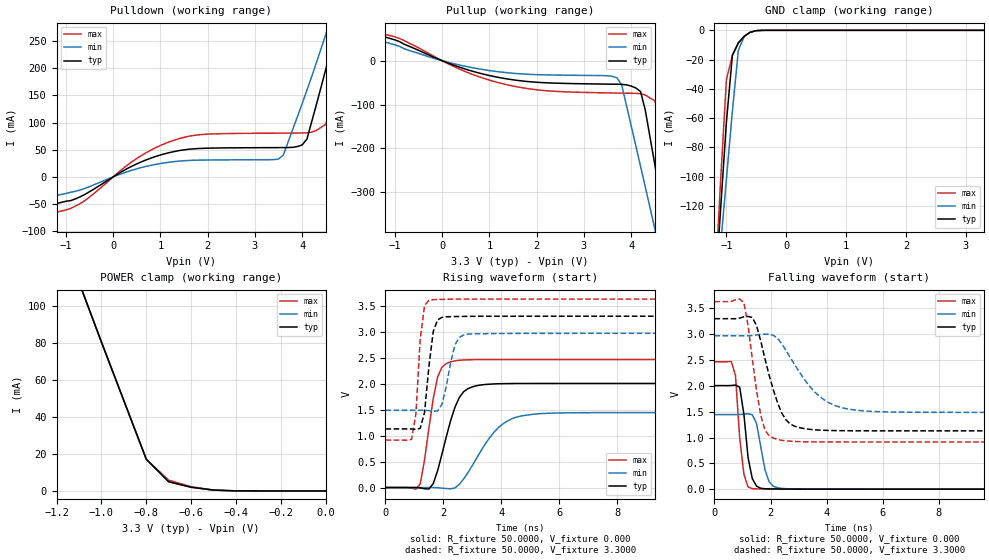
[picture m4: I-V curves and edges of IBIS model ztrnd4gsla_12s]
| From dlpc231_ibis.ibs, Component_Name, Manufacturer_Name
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| Model ztrnd4gsla_12s
[Model]   ztrnd4gsla_12s
Model_type   I/O
Polarity   Non-Inverting
Enable   Active-High
Vinl = 0.8000V
Vinh = 2.0000V
Vmeas = 1.5000V
Cref =50.0000pF
Rref = 0.5000k
Vref =  0.000V
C_comp   0.7000pF   0.7000pF   0.7000pF
[Temperature Range]   25.0000   0.1240k   -40.0000
[Voltage Range]   3.3000V   2.9700V   3.6300V
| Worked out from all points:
|   slope of the pulldown table from 0 to 0.495 V, typ, clamps not added: 20.8 ohm
|   slope of the pullup table from 0 to 0.495 V, typ, clamps not added: 25.7 ohm
|   GND clamp passes 1 mA (typ) near -0.57 V on its own axis
|   POWER clamp passes 1 mA (typ) near -0.54 V on its own axis
|   rising waveform, R_fixture 50.0000, V_fixture 0.000: 20-80 % time 609ps typ, 1.05ns min, 408ps max; typ from 0 V to 2 V
|   rising waveform, R_fixture 50.0000, V_fixture 3.3000: 20-80 % time 249ps typ, 339ps min, 199ps max; typ from 1.13 V to 3.3 V
|   falling waveform, R_fixture 50.0000, V_fixture 0.000: 20-80 % time 270ps typ, 317ps min, 228ps max; typ from 2 V to 0 V
|   falling waveform, R_fixture 50.0000, V_fixture 3.3000: 20-80 % time 681ps typ, 1.22ns min, 426ps max; typ from 3.3 V to 1.13 V
[Pulldown]
-3.3V     -73mA      -55mA      -90mA
-900mV    -43.69mA   -28.26mA   -58.09mA
500mV     23.99mA    14.89mA    33.9mA
1.4V      48.44mA    29.06mA    70.56mA
3.5V      53.88mA    32.86mA    80.51mA
3.6V      53.91mA    40.18mA    80.55mA
4.1V      69.56mA    159.6mA    81.03mA
4.5V      198.3mA    262.5mA    96.9mA
4.7V      266mA      317.2mA    172.7mA
4.9V      336.1mA    374.9mA    257.2mA
5.1V      409.2mA    436.3mA    344.5mA
6.6V      1.092A     994.6mA    1.119A
[Pullup]
-3.3V     43mA       55.7mA     31mA
-2.5V     69.3mA     66.1mA     65.5mA
-1.5V     63.3mA     51.6mA     67.9mA
1.2V      -38.25mA   -25.31mA   -50.33mA
3.7V      -53.69mA   -39.1mA    -73.83mA
3.8V      -53.99mA   -55.36mA   -73.99mA
4.2V      -70.44mA   -241.6mA   -75.38mA
4.5V      -236.8mA   -383.2mA   -91.7mA
4.7V      -361.3mA   -478.4mA   -150.8mA
4.9V      -486.6mA   -574.2mA   -307mA
5.1V      -612.6mA   -670.5mA   -464.3mA
6.6V      -1.569A    -1.403A    -1.657A
[GND_clamp]
-3.3V     -1.517A    -1.206A    -1.849A
-1.2V     -185.7mA   -194.8mA   -182.8mA
-1.1V     -124mA     -148.1mA   -104.8mA
-1V       -62.54mA   -101.7mA   -33.61mA
-900mV    -17.04mA   -55.16mA   -17.04mA
-800mV    -8.525mA   -13.45mA   -8.525mA
-700mV    -3.999mA   -3.999mA   -3.999mA
-600mV    -1.289mA   -1.289mA   -1.289mA
-500mV    -219.7uA   -252.6uA   -203.6uA
-400mV    -15.61uA   -27.49uA   -11.15uA
3.3V      3.373nA    3.373nA    17.05nA
[POWER_clamp]
-3.3V     1.027A     840.1mA    1.22A
-1.1V     112.7mA    112.7mA    112.7mA
-1V       80.41mA    80.41mA    80.41mA
-800mV    17.08mA    17.08mA    17.08mA
-700mV    4.947mA    4.947mA    5.794mA
-600mV    1.98mA     1.98mA     2.27mA
-500mV    443.8uA    443.8uA    443.8uA
-400mV    34.78uA    34.78uA    34.78uA
0V        3.373nA    3.373nA    57.43nA
[Ramp]
dV/dt_r   1.2030/0.6030n   0.8658/1.0497n   1.4790/0.3987n
dV/dt_f   1.3026/0.6787n   0.8892/1.2110n   1.6300/0.4288n
R_load = 50.0000
[Rising Waveform]
R_fixture = 50.0000
V_fixture = 0.000
V_fixture_min = 0.000
V_fixture_max = 0.000
0s        0V         0V         0V
1.2ns     -7.803mV   -9.584uV   71.28mV
1.5ns     -27.26mV   606uV      1.148V
1.8ns     323.8mV    -3.174mV   2.128V
2.25ns    1.289V     -23.92mV   2.422V
2.55ns    1.735V     62.9mV     2.451V
2.85ns    1.905V     287.9mV    2.46V
3.75ns    1.996V     1.068V     2.465V
4.65ns    2.004V     1.374V     2.465V
14.85ns   2.005V     1.443V     2.465V
[Rising Waveform]
R_fixture = 50.0000
V_fixture = 3.3000
V_fixture_min = 2.9700
V_fixture_max = 3.6300
0s        1.129V     1.487V     913.4mV
900ps     1.129V     1.487V     928mV
1.05ns    1.12V      1.487V     1.421V
1.2ns     1.14V      1.487V     2.86V
1.35ns    1.45V      1.487V     3.507V
1.5ns     2.336V     1.482V     3.606V
1.8ns     3.229V     1.477V     3.621V
2.4ns     3.293V     2.749V     3.628V
2.7ns     3.296V     2.939V     3.629V
14.85ns   3.3V       2.97V      3.63V
[Falling Waveform]
R_fixture = 50.0000
V_fixture = 0.000
V_fixture_min = 0.000
V_fixture_max = 0.000
0s        2.005V     1.443V     2.465V
600ps     2.007V     1.443V     2.471V
750ps     2.015V     1.443V     2.202V
900ps     1.974V     1.444V     989mV
1.05ns    1.45V      1.451V     291mV
1.2ns     603.7mV    1.46V      40.83mV
1.35ns    203.2mV    1.44V      10.11mV
1.95ns    5.931mV    140.7mV    3.047mV
2.25ns    4.213mV    27.31mV    1.571mV
14.85ns   0V         0V         0V
[Falling Waveform]
R_fixture = 50.0000
V_fixture = 3.3000
V_fixture_min = 2.9700
V_fixture_max = 3.6300
0s        3.3V       2.97V      3.63V
1.05ns    3.336V     2.969V     3.612V
1.35ns    3.324V     2.974V     2.519V
1.65ns    2.869V     2.999V     1.435V
1.8ns     2.526V     3.001V     1.143V
2.1ns     1.921V     2.979V     988.7mV
2.7ns     1.262V     2.551V     928.4mV
3.6ns     1.148V     1.867V     914.9mV
4.65ns    1.132V     1.563V     913.5mV
14.85ns   1.129V     1.487V     913.4mV
